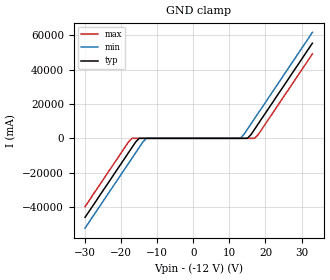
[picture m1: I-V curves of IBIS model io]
| TEXAS INSTRUMENTS INCORPORATED
| 2 Channel-Bi-directional ESD Protection Device
| Marketing Part #   Voltage Range   Package-type   #pins/pkg drawing
| ESD862   -12V-12V   SOT   3/DBZ
[IBIS Ver]   4.1
[Comment char]  |_char
[File Name]   esd562.ibs
[File Rev]   1.0
"[Date]   Jan 15, 2024 "
[Source]   Data created from TI-SPICE simulations at TI-SLL/HVL.
   The following is an IBIS list for the ESD562.
   Please contact sllibis@ti.com with questions and
   comments concerning SLL IBIS models.
[Notes]
   - New measurements under nominal conditions only.
[Disclaimer]
"| TI and its licensors and suppliers make no warranties, either expressed"
"| or implied, with respect to this  model, including the warranties of "
"| provided solely on an ""as is"" basis. The entire risk as to its quality "
| and performance is with the customer.
[Copyright]
| (C) Copyright 2024 Texas Instruments Incorporated. All rights reserved.
| Component ESD562_DBZ 3-PIN SOT
[Component]   ESD562_DBZ
"[Manufacturer]   Texas Instruments, Inc."
[Package]   |3 SOT - DBZ package
   typ   min   max
R_pkg   10.3E-02   5.3E-02   15.3E-02
L_pkg   1.84E-10   0.8E-10   2.6E-10
C_pkg   2.3E-13   1.3E-13   3.3E-13
[Pin]   signal_name   model_name   R_pin   L_pin   C_pin
1   IO   io   2.07E-03   2.09E-10   6.95E-14
2   IO   io   2.07E-03   2.09E-10   6.95E-14
3   GND   gnd   2.07E-03   2.09E-10   6.95E-14
| Models and submodels in the file (1): io (Input)
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|   io Model
[Model]   io
Model_type  Input
| variable   typ   min   max
C_comp   1.5pF   1.1pF   1.9pF
[Voltage Range]   24   20   28
[Temperature Range]   27   -55   150
[Power Clamp Reference]   0   0   0
[GND Clamp Reference]   -12   -10   -14
[GND Clamp]
|	Voltage  I(typ)   I(min)   I(max)
-30V      -45.9A     -52.2A     -39.7A
-18V      -8.44A     -14.7A     -2.19A
-17V      -5.31A     -11.6A     -11.1nA
-16V      -2.19A     -8.44A     -10.5nA
-15V      -9.8nA     -5.31A     -9.8nA
-13V      -8.5nA     -8.5nA     -8.5nA
13V       8.5nA      8.5nA      8.5nA
15V       9.8nA      5.31A      9.8nA
16V       2.19A      8.44A      10.5nA
17V       5.31A      11.6A      11.1nA
18V       8.44A      14.7A      2.19A
33V       55.3A      61.6A      49.1A
[Power Clamp]
|   Voltage   I(typ)   I(min)   I(max)
-12V      0A         0A         0A
0V        0A         0A         0A
12V       0A         0A         0A
